(* Logix 5000 Program export KEP; software revision 30.00; part 15 of 15 *)
(* tags used below, declared in another part *)
   B256_CtoE : B256_CtoE;
   B256_EtoDINT : B256_EtoDINT;
   B256_EtoL : B256_EtoL;
   B256_StoC : B256_StoC;
   B256_StoC_LE : B256_StoC_LE;
   EdDSA_INTERNAL : EdDSA_INTERNAL[5];
   EdDSA_STATES : EdDSA_STATECTRL[15];
   InternalFlags : InternalFlags[5];
   InternalFlag_KsExists : BOOL;
   POINT_DEC : POINT_DEC;
   POINT_ENC : POINT_ENC;
   POINT_MUL : POINT_MUL;
   ServerNode : INT;
   SHA512_SEQ : SHA512_SEQ;
   Temp_Processor_C1 : DINT[22];
   Temp_Processor_C10 : DINT[22];
   Temp_Processor_C11 : DINT[22];
   Temp_Processor_C12 : DINT[22];
   Temp_Processor_C2 : DINT[22];
   Temp_Processor_C3 : DINT[22];
   Temp_Processor_C4 : DINT[22];
   Temp_Processor_C5 : DINT[22];
   Temp_Processor_C6 : DINT[22];
   Temp_Processor_C7 : DINT[22];
   Temp_Processor_C8 : DINT[22];
   Temp_Processor_C9 : DINT[22];
   Temp_Processor_D1 : DINT[43];
   Temp_Processor_DINT1 : DINT[8];
   Temp_Processor_DINT2 : DINT[8];
   Temp_Processor_E1 : DINT[32];
   Temp_Processor_E2 : DINT[32];
   Temp_Processor_HASH : LINT[8];
   Temp_Processor_L : LINT[4];
   Temp_Processor_MSG : LINT[1600];
   Temp_Processor_P1 : POINT;
   Temp_Processor_P2 : POINT;
   Temp_Processor_P3 : POINT;
   Temp_Processor_P4 : POINT;
   T_INT1 : INT;
   EdDSA_KS_Prime : DINT[8];
   InternalFlag_KsPrimeID : LINT;
   Wrk_InpA : DINT[2];
(* KEP, continued *)

ROUTINE PROCESSOR_STATE9   (* ladder *)
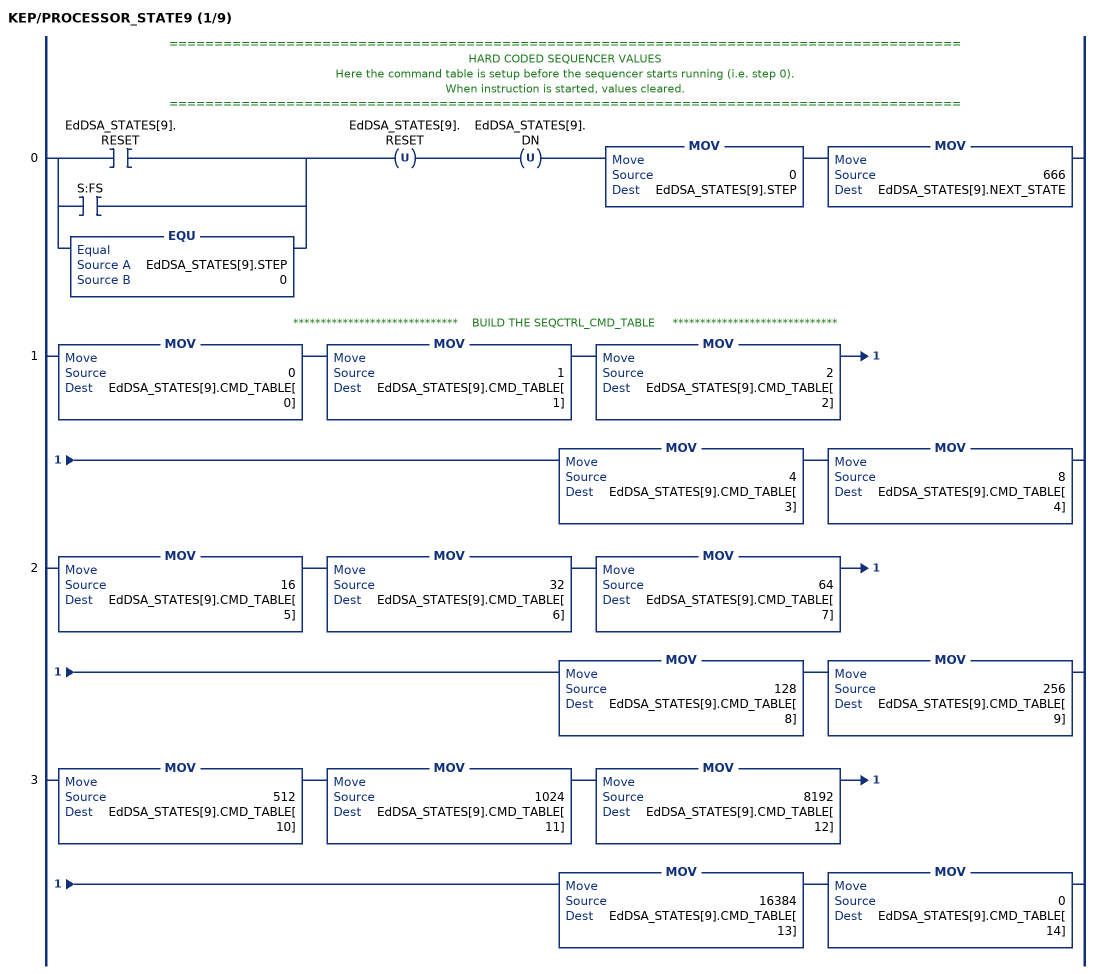
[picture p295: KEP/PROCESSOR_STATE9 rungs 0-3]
   // ========================================================================================
   // HARD CODED SEQUENCER VALUES
   // Here the command table is setup before the sequencer starts running (i.e. step 0).
   // When instruction is started, values cleared.
   // ========================================================================================
   0: [[XIC(EdDSA_STATES[9].RESET) ,XIC(S:FS) ] ,EQU(EdDSA_STATES[9].STEP,0) ]OTU(EdDSA_STATES[9].RESET)OTU(EdDSA_STATES[9].DN)MOV(0,EdDSA_STATES[9].STEP)MOV(666,EdDSA_STATES[9].NEXT_STATE);
   // ******************************    BUILD THE SEQCTRL_CMD_TABLE     ******************************
   1: MOV(0,EdDSA_STATES[9].CMD_TABLE[0])MOV(1,EdDSA_STATES[9].CMD_TABLE[1])MOV(2,EdDSA_STATES[9].CMD_TABLE[2])MOV(4,EdDSA_STATES[9].CMD_TABLE[3])MOV(8,EdDSA_STATES[9].CMD_TABLE[4]);
   2: MOV(16,EdDSA_STATES[9].CMD_TABLE[5])MOV(32,EdDSA_STATES[9].CMD_TABLE[6])MOV(64,EdDSA_STATES[9].CMD_TABLE[7])MOV(128,EdDSA_STATES[9].CMD_TABLE[8])MOV(256,EdDSA_STATES[9].CMD_TABLE[9]);
   3: MOV(512,EdDSA_STATES[9].CMD_TABLE[10])MOV(1024,EdDSA_STATES[9].CMD_TABLE[11])MOV(8192,EdDSA_STATES[9].CMD_TABLE[12])MOV(16384,EdDSA_STATES[9].CMD_TABLE[13])MOV(0,EdDSA_STATES[9].CMD_TABLE[14]);
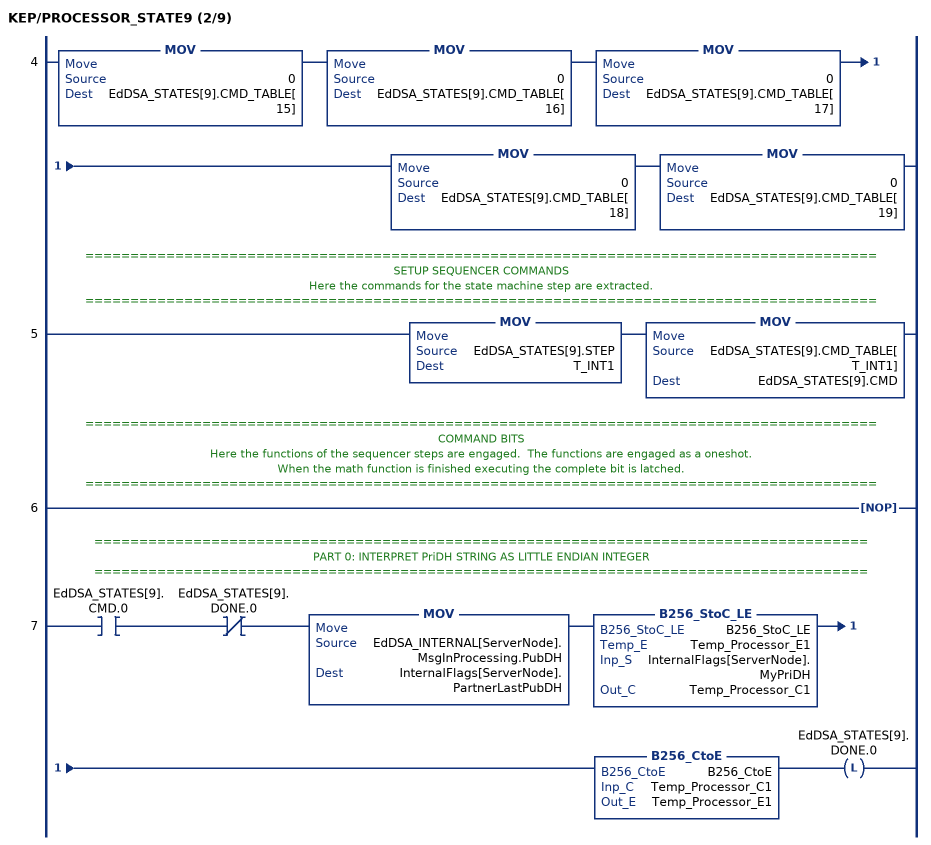
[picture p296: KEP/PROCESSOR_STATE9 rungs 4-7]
   4: MOV(0,EdDSA_STATES[9].CMD_TABLE[15])MOV(0,EdDSA_STATES[9].CMD_TABLE[16])MOV(0,EdDSA_STATES[9].CMD_TABLE[17])MOV(0,EdDSA_STATES[9].CMD_TABLE[18])MOV(0,EdDSA_STATES[9].CMD_TABLE[19]);
   // ========================================================================================
   // SETUP SEQUENCER COMMANDS
   // Here the commands for the state machine step are extracted.
   // ========================================================================================
   5: MOV(EdDSA_STATES[9].STEP,T_INT1)MOV(EdDSA_STATES[9].CMD_TABLE[T_INT1],EdDSA_STATES[9].CMD);
   // ========================================================================================
   // COMMAND BITS
   // Here the functions of the sequencer steps are engaged.  The functions are engaged as a oneshot.
   // When the math function is finished executing the complete bit is latched.
   // ========================================================================================
   6: NOP();
   // ======================================================================================
   // PART 0: INTERPRET PriDH STRING AS LITTLE ENDIAN INTEGER
   // ======================================================================================
   7: XIC(EdDSA_STATES[9].CMD.0)XIO(EdDSA_STATES[9].DONE.0)MOV(EdDSA_INTERNAL[ServerNode].MsgInProcessing.PubDH,InternalFlags[ServerNode].PartnerLastPubDH)B256_StoC_LE(B256_StoC_LE,Temp_Processor_E1,InternalFlags[ServerNode].MyPriDH,Temp_Processor_C1)B256_CtoE(B256_CtoE,Temp_Processor_C1,Temp_Processor_E1)OTL(EdDSA_STATES[9].DONE.0);
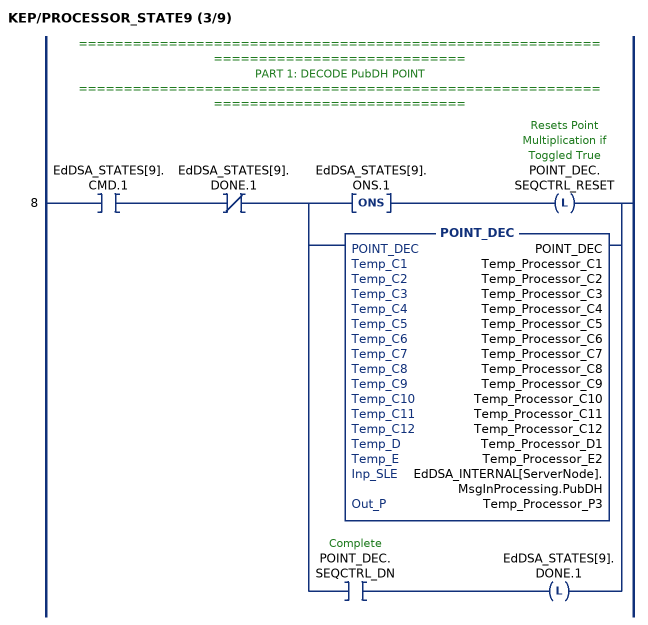
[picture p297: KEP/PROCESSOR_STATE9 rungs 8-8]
   // ======================================================================================
   // PART 1: DECODE PubDH POINT
   // ======================================================================================
   8: XIC(EdDSA_STATES[9].CMD.1)XIO(EdDSA_STATES[9].DONE.1)[ONS(EdDSA_STATES[9].ONS.1) OTL(POINT_DEC.SEQCTRL_RESET) ,POINT_DEC(POINT_DEC,Temp_Processor_C1,Temp_Processor_C2,Temp_Processor_C3,Temp_Processor_C4,Temp_Processor_C5,Temp_Processor_C6,Temp_Processor_C7,Temp_Processor_C8,Temp_Processor_C9,Temp_Processor_C10,Temp_Processor_C11,Temp_Processor_C12,Temp_Processor_D1,Temp_Processor_E2,EdDSA_INTERNAL[ServerNode].MsgInProcessing.PubDH,Temp_Processor_P3) ,XIC(POINT_DEC.SEQCTRL_DN) OTL(EdDSA_STATES[9].DONE.1) ];
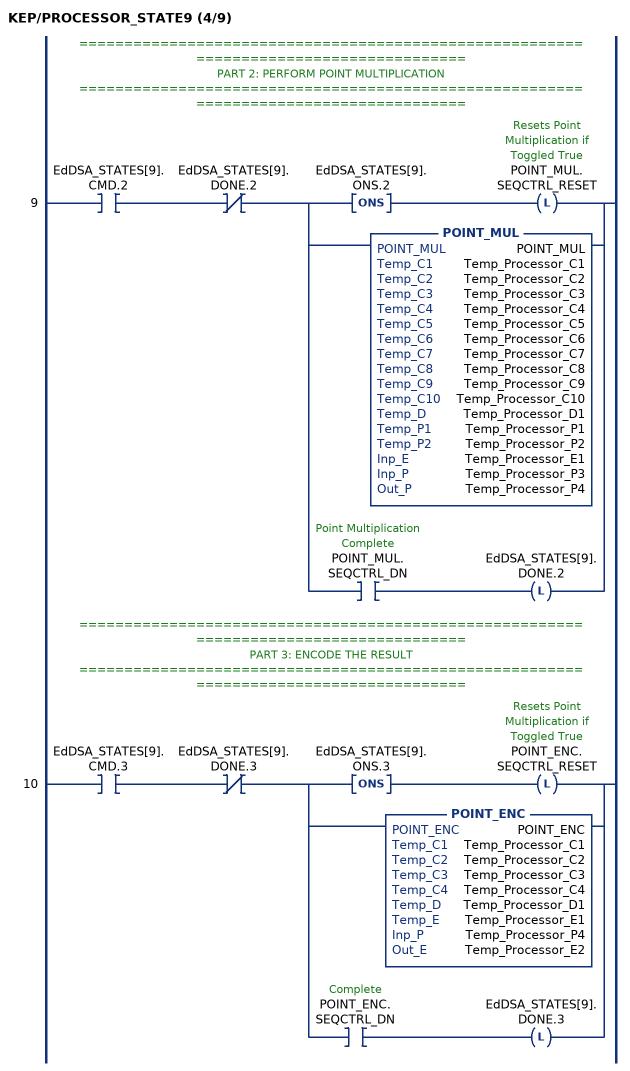
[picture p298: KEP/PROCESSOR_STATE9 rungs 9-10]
   // ======================================================================================
   // PART 2: PERFORM POINT MULTIPLICATION
   // ======================================================================================
   9: XIC(EdDSA_STATES[9].CMD.2)XIO(EdDSA_STATES[9].DONE.2)[ONS(EdDSA_STATES[9].ONS.2) OTL(POINT_MUL.SEQCTRL_RESET) ,POINT_MUL(POINT_MUL,Temp_Processor_C1,Temp_Processor_C2,Temp_Processor_C3,Temp_Processor_C4,Temp_Processor_C5,Temp_Processor_C6,Temp_Processor_C7,Temp_Processor_C8,Temp_Processor_C9,Temp_Processor_C10,Temp_Processor_D1,Temp_Processor_P1,Temp_Processor_P2,Temp_Processor_E1,Temp_Processor_P3,Temp_Processor_P4) ,XIC(POINT_MUL.SEQCTRL_DN) OTL(EdDSA_STATES[9].DONE.2) ];
   // ======================================================================================
   // PART 3: ENCODE THE RESULT
   // ======================================================================================
   10: XIC(EdDSA_STATES[9].CMD.3)XIO(EdDSA_STATES[9].DONE.3)[ONS(EdDSA_STATES[9].ONS.3) OTL(POINT_ENC.SEQCTRL_RESET) ,POINT_ENC(POINT_ENC,Temp_Processor_C1,Temp_Processor_C2,Temp_Processor_C3,Temp_Processor_C4,Temp_Processor_D1,Temp_Processor_E1,Temp_Processor_P4,Temp_Processor_E2) ,XIC(POINT_ENC.SEQCTRL_DN) OTL(EdDSA_STATES[9].DONE.3) ];
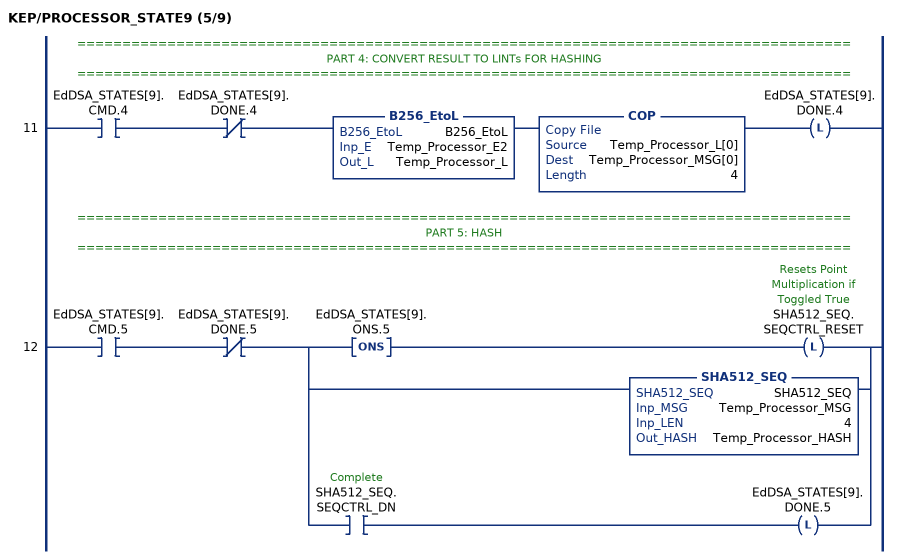
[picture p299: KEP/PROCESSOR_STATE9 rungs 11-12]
   // ======================================================================================
   // PART 4: CONVERT RESULT TO LINTs FOR HASHING
   // ======================================================================================
   11: XIC(EdDSA_STATES[9].CMD.4)XIO(EdDSA_STATES[9].DONE.4)B256_EtoL(B256_EtoL,Temp_Processor_E2,Temp_Processor_L)COP(Temp_Processor_L[0],Temp_Processor_MSG[0],4)OTL(EdDSA_STATES[9].DONE.4);
   // ======================================================================================
   // PART 5: HASH
   // ======================================================================================
   12: XIC(EdDSA_STATES[9].CMD.5)XIO(EdDSA_STATES[9].DONE.5)[ONS(EdDSA_STATES[9].ONS.5) OTL(SHA512_SEQ.SEQCTRL_RESET) ,SHA512_SEQ(SHA512_SEQ,Temp_Processor_MSG,4,Temp_Processor_HASH) ,XIC(SHA512_SEQ.SEQCTRL_DN) OTL(EdDSA_STATES[9].DONE.5) ];
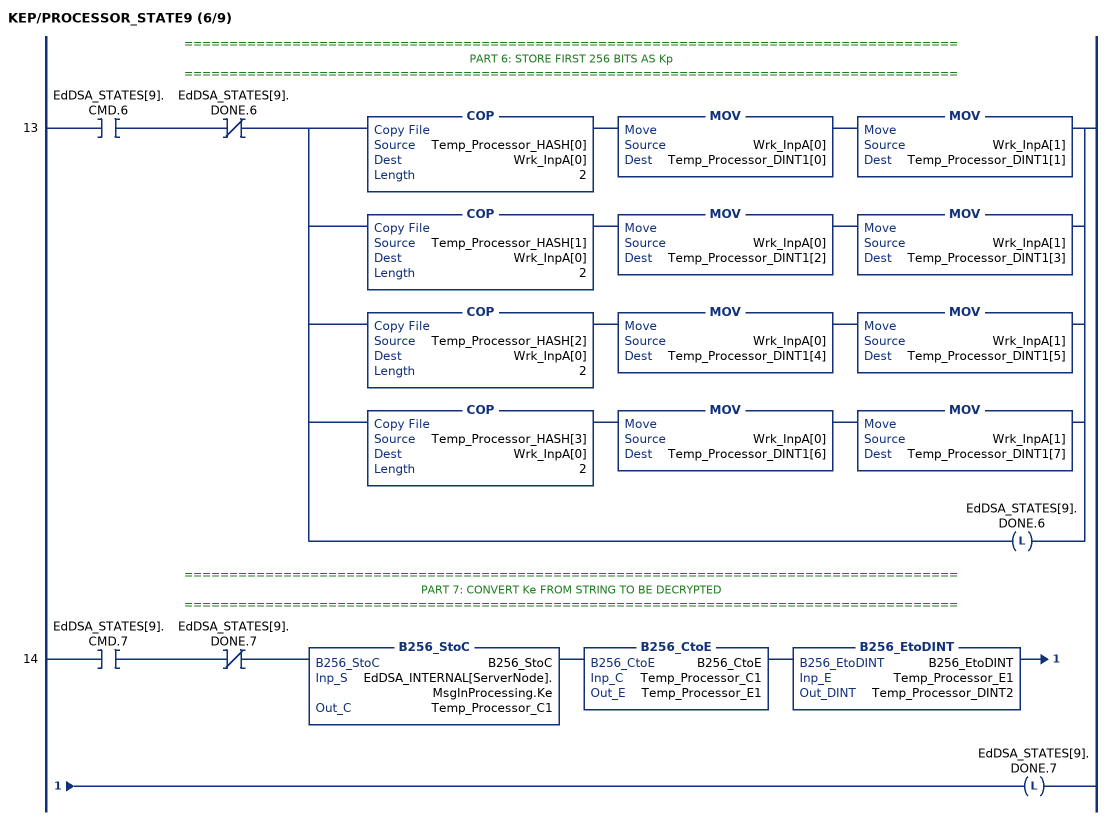
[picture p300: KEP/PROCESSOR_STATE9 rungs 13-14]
   // ======================================================================================
   // PART 6: STORE FIRST 256 BITS AS Kp
   // ======================================================================================
   13: XIC(EdDSA_STATES[9].CMD.6)XIO(EdDSA_STATES[9].DONE.6)[COP(Temp_Processor_HASH[0],Wrk_InpA[0],2) MOV(Wrk_InpA[0],Temp_Processor_DINT1[0]) MOV(Wrk_InpA[1],Temp_Processor_DINT1[1]) ,COP(Temp_Processor_HASH[1],Wrk_InpA[0],2) MOV(Wrk_InpA[0],Temp_Processor_DINT1[2]) MOV(Wrk_InpA[1],Temp_Processor_DINT1[3]) ,COP(Temp_Processor_HASH[2],Wrk_InpA[0],2) MOV(Wrk_InpA[0],Temp_Processor_DINT1[4]) MOV(Wrk_InpA[1],Temp_Processor_DINT1[5]) ,COP(Temp_Processor_HASH[3],Wrk_InpA[0],2) MOV(Wrk_InpA[0],Temp_Processor_DINT1[6]) MOV(Wrk_InpA[1],Temp_Processor_DINT1[7]) ,OTL(EdDSA_STATES[9].DONE.6) ];
   // ======================================================================================
   // PART 7: CONVERT Ke FROM STRING TO BE DECRYPTED
   // ======================================================================================
   14: XIC(EdDSA_STATES[9].CMD.7)XIO(EdDSA_STATES[9].DONE.7)B256_StoC(B256_StoC,EdDSA_INTERNAL[ServerNode].MsgInProcessing.Ke,Temp_Processor_C1)B256_CtoE(B256_CtoE,Temp_Processor_C1,Temp_Processor_E1)B256_EtoDINT(B256_EtoDINT,Temp_Processor_E1,Temp_Processor_DINT2)OTL(EdDSA_STATES[9].DONE.7);
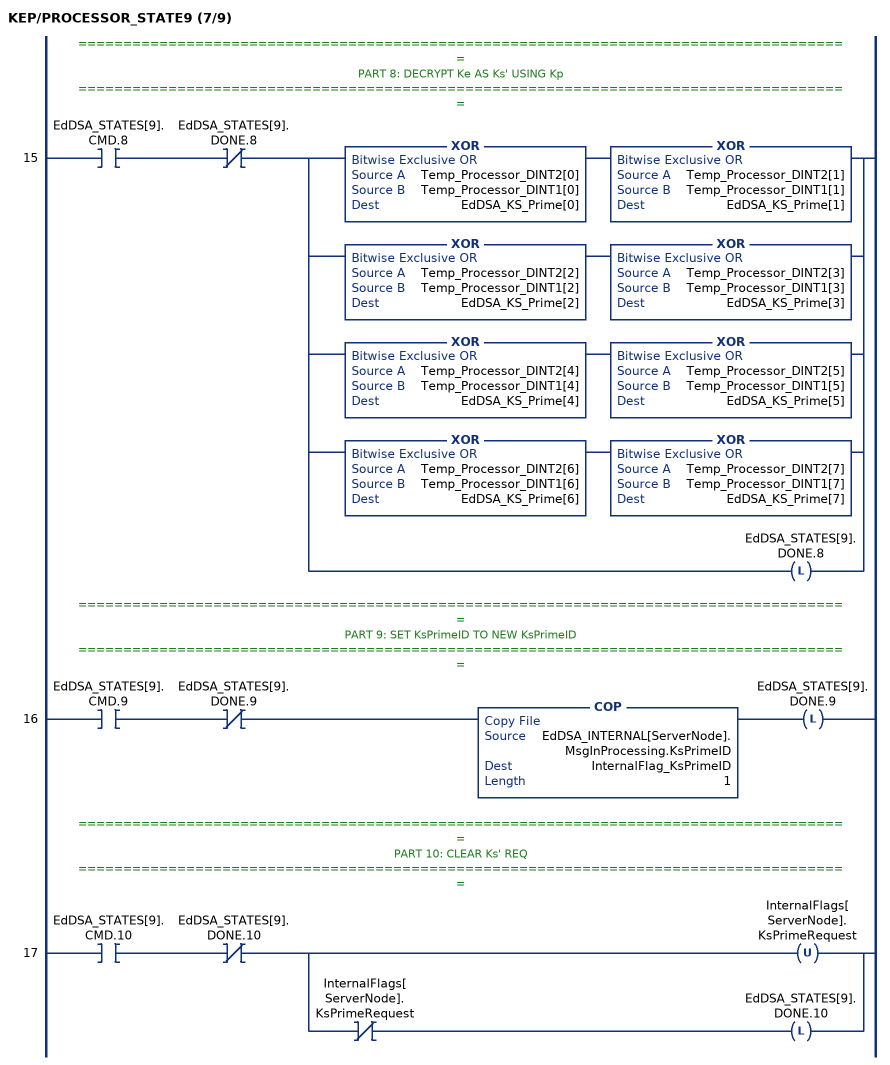
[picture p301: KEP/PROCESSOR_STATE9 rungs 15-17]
   // ======================================================================================
   // PART 8: DECRYPT Ke AS Ks' USING Kp
   // ======================================================================================
   15: XIC(EdDSA_STATES[9].CMD.8)XIO(EdDSA_STATES[9].DONE.8)[XOR(Temp_Processor_DINT2[0],Temp_Processor_DINT1[0],EdDSA_KS_Prime[0]) XOR(Temp_Processor_DINT2[1],Temp_Processor_DINT1[1],EdDSA_KS_Prime[1]) ,XOR(Temp_Processor_DINT2[2],Temp_Processor_DINT1[2],EdDSA_KS_Prime[2]) XOR(Temp_Processor_DINT2[3],Temp_Processor_DINT1[3],EdDSA_KS_Prime[3]) ,XOR(Temp_Processor_DINT2[4],Temp_Processor_DINT1[4],EdDSA_KS_Prime[4]) XOR(Temp_Processor_DINT2[5],Temp_Processor_DINT1[5],EdDSA_KS_Prime[5]) ,XOR(Temp_Processor_DINT2[6],Temp_Processor_DINT1[6],EdDSA_KS_Prime[6]) XOR(Temp_Processor_DINT2[7],Temp_Processor_DINT1[7],EdDSA_KS_Prime[7]) ,OTL(EdDSA_STATES[9].DONE.8) ];
   // ======================================================================================
   // PART 9: SET KsPrimeID TO NEW KsPrimeID
   // ======================================================================================
   16: XIC(EdDSA_STATES[9].CMD.9)XIO(EdDSA_STATES[9].DONE.9)COP(EdDSA_INTERNAL[ServerNode].MsgInProcessing.KsPrimeID,InternalFlag_KsPrimeID,1)OTL(EdDSA_STATES[9].DONE.9);
   // ======================================================================================
   // PART 10: CLEAR Ks' REQ
   // ======================================================================================
   17: XIC(EdDSA_STATES[9].CMD.10)XIO(EdDSA_STATES[9].DONE.10)[OTU(InternalFlags[ServerNode].KsPrimeRequest) ,XIO(InternalFlags[ServerNode].KsPrimeRequest) OTL(EdDSA_STATES[9].DONE.10) ];
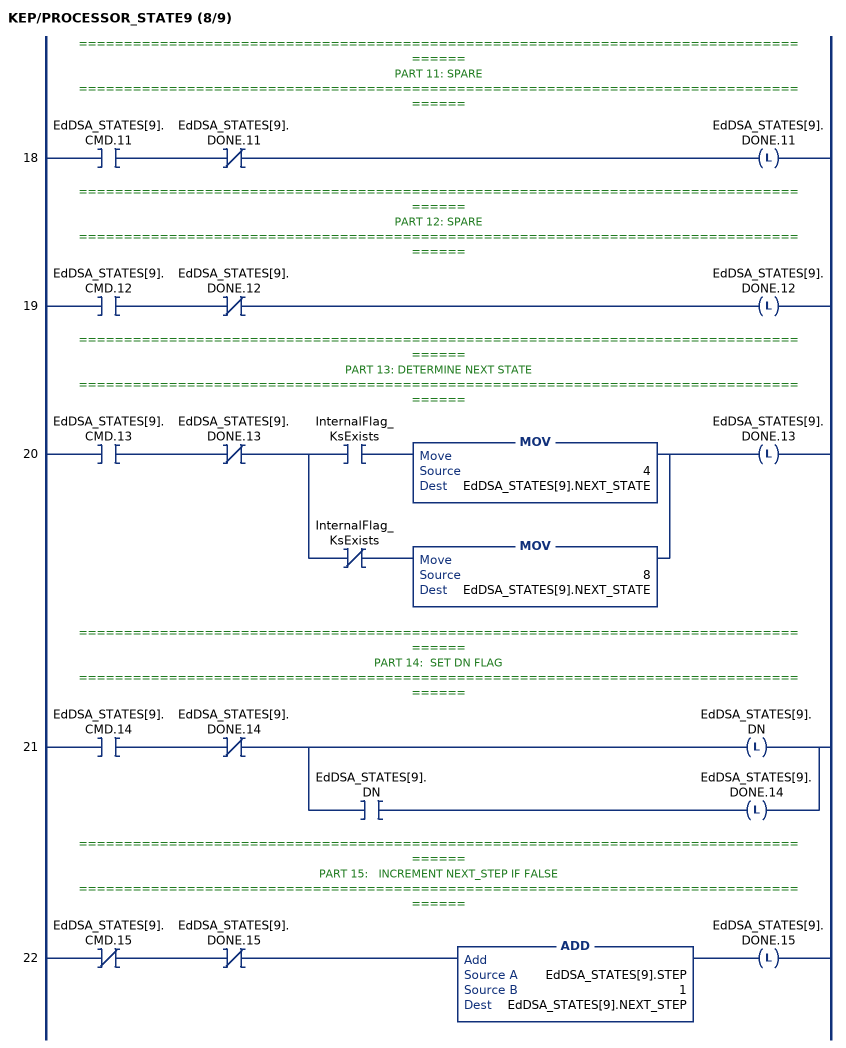
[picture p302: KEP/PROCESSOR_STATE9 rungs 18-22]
   // ======================================================================================
   // PART 11: SPARE
   // ======================================================================================
   18: XIC(EdDSA_STATES[9].CMD.11)XIO(EdDSA_STATES[9].DONE.11)OTL(EdDSA_STATES[9].DONE.11);
   // ======================================================================================
   // PART 12: SPARE
   // ======================================================================================
   19: XIC(EdDSA_STATES[9].CMD.12)XIO(EdDSA_STATES[9].DONE.12)OTL(EdDSA_STATES[9].DONE.12);
   // ======================================================================================
   // PART 13: DETERMINE NEXT STATE
   // ======================================================================================
   20: XIC(EdDSA_STATES[9].CMD.13)XIO(EdDSA_STATES[9].DONE.13)[XIC(InternalFlag_KsExists) MOV(4,EdDSA_STATES[9].NEXT_STATE) ,XIO(InternalFlag_KsExists) MOV(8,EdDSA_STATES[9].NEXT_STATE) ]OTL(EdDSA_STATES[9].DONE.13);
   // ======================================================================================
   // PART 14:  SET DN FLAG
   // ======================================================================================
   21: XIC(EdDSA_STATES[9].CMD.14)XIO(EdDSA_STATES[9].DONE.14)[OTL(EdDSA_STATES[9].DN) ,XIC(EdDSA_STATES[9].DN) OTL(EdDSA_STATES[9].DONE.14) ];
   // ======================================================================================
   // PART 15:   INCREMENT NEXT_STEP IF FALSE
   // ======================================================================================
   22: XIO(EdDSA_STATES[9].CMD.15)XIO(EdDSA_STATES[9].DONE.15)ADD(EdDSA_STATES[9].STEP,1,EdDSA_STATES[9].NEXT_STEP)OTL(EdDSA_STATES[9].DONE.15);
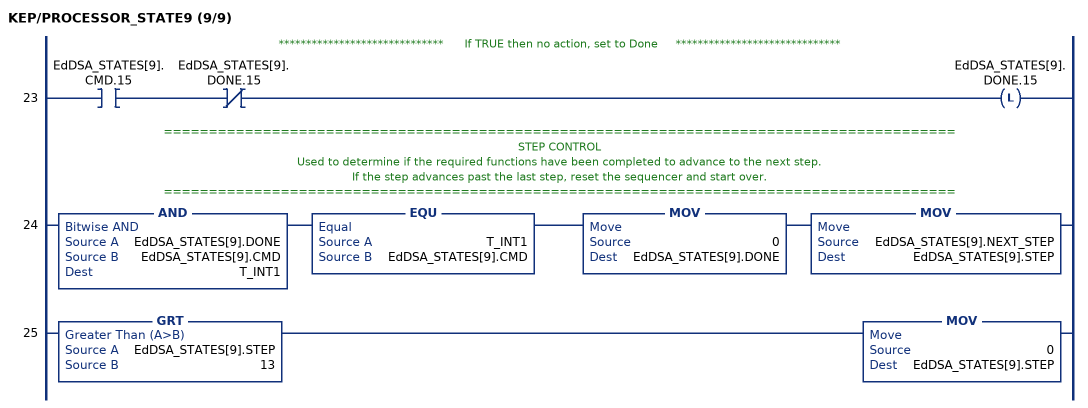
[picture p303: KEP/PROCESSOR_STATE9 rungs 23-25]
   // ******************************      If TRUE then no action, set to Done     ******************************
   23: XIC(EdDSA_STATES[9].CMD.15)XIO(EdDSA_STATES[9].DONE.15)OTL(EdDSA_STATES[9].DONE.15);
   // ========================================================================================
   // STEP CONTROL
   // Used to determine if the required functions have been completed to advance to the next step.
   // If the step advances past the last step, reset the sequencer and start over.
   // ========================================================================================
   24: AND(EdDSA_STATES[9].DONE,EdDSA_STATES[9].CMD,T_INT1)EQU(T_INT1,EdDSA_STATES[9].CMD)MOV(0,EdDSA_STATES[9].DONE)MOV(EdDSA_STATES[9].NEXT_STEP,EdDSA_STATES[9].STEP);
   25: GRT(EdDSA_STATES[9].STEP,13)MOV(0,EdDSA_STATES[9].STEP);
END_ROUTINE
END_PROGRAM
